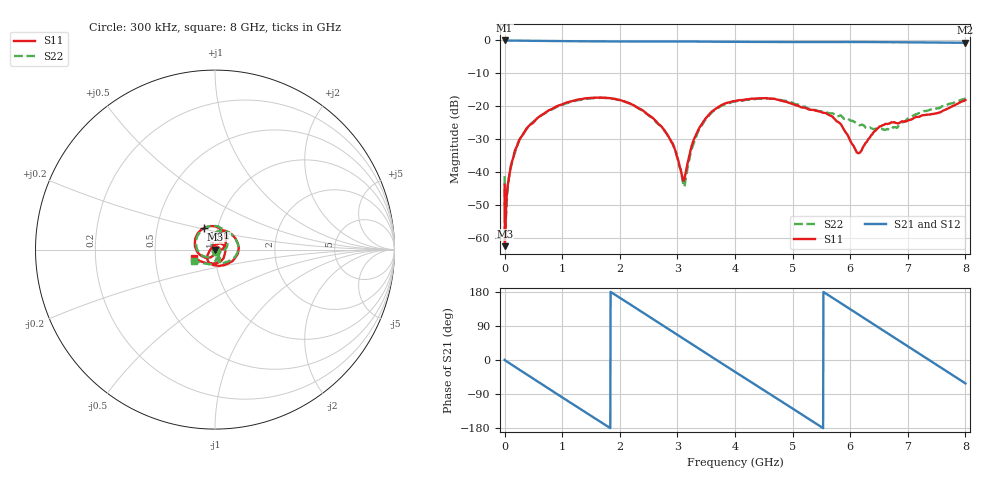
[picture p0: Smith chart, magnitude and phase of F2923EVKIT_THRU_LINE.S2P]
! Integrated Device Technology
! Corporate Headquarters
! 6024 Silver Creek Valley Road
! San Jose, CA 95138  USA
! Phone:  1-408-284-8200
! Toll Free:  1-800-223-1366
! Webpage:  http://www.idt.com/
! Timing and RF Division
! 515 Groton Road, Suite 102
! Westford, MA 01886-6024
! Description: F2923 EVKIT Thru Line
! Frequency:  0.3 MHz to 8 GHz
! Ports:  2 RF, 0 DC
!  EVKit RF Connector J4  = Port 1
!  EVKit RF Connector J5  = Port 2
! Data:  The results below were measured on the F2923 EVKit Thru Line from J4 to J5
!  using a calibrated network analyzer. The reference plane is at
!  the SMA coaxial interfaces.
! Misc:
! Date Measured:  2017-08-14
! Date:  2017-08-14  SPJ
! Note:
!  Integrated Device Technology supplies this data as a sample
!	of measured data. Data was taken at 25 degrees C.
!  Integrated Device Technology reserves the right to change
! 	this data at anytime.
# Hz S dB R 50
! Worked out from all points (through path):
!   1601 points, 300 kHz to 8 GHz, reference 50 ohm
!   highest |S21| = 0.01 dB at 300 kHz (marker M1); lowest = -0.7 dB at 8 GHz (marker M2)
!   group delay of S21, straight-line fit = 271 ps
!   lowest |S11| = -62.6 dB at 5.3 MHz (marker M3), VSWR 1.00, Z = 50.1 - j0.02 ohm
!   |S11| at or under -10 dB: start of sweep to end of sweep
!   |S22| runs from -59.3 to -17.4 dB; largest |S21 - S12| = 0.0061
!   S11 on the Smith chart (normalised r, x): 300 kHz: 1.01, -0.01; 1.61 GHz: 0.86, +0.21; 8 GHz: 0.79, -0.07
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300000  -43.92 -40.7  0.01 0.2  -0.00 0.2  -41.32 -48.5
5299813  -62.63 -15.7  0.00 -0.6  0.00 -0.6  -59.33 55.5
4.529831e7  -45.58 -62.4  -0.01 -4.6  -0.02 -4.6  -46.56 -73.0
9.029662e7  -40.40 -77.5  -0.02 -9.1  -0.03 -9.1  -40.13 -80.4
1.652938e8  -34.50 -88.0  -0.04 -16.6  -0.04 -16.6  -34.82 -95.3
3.952852e8  -26.50 -116.7  -0.08 -39.3  -0.08 -39.3  -26.56 -121.1
8.652676e8  -20.45 -167.9  -0.16 -85.4  -0.16 -85.4  -20.63 -173.9
1.33525e9  -17.88 144.9  -0.24 -131.2  -0.25 -131.2  -17.99 136.4
1.61024e9  -17.39 118.0  -0.27 -157.9  -0.28 -157.9  -17.52 108.9
2.100221e9  -18.71 71.9  -0.29 154.6  -0.29 154.5  -18.73 62.4
2.6702e9  -25.40 16.3  -0.28 99.0  -0.28 99.0  -25.51 -3.5
2.93519e9  -32.22 -3.5  -0.29 73.0  -0.29 73.1  -32.09 -42.9
3.115183e9  -42.53 63.6  -0.30 55.4  -0.30 55.4  -44.56 -138.5
3.440171e9  -24.97 102.1  -0.34 23.5  -0.33 23.5  -25.33 110.4
4.00015e9  -18.43 59.9  -0.41 -31.2  -0.41 -31.1  -18.59 61.7
4.655125e9  -17.74 -7.9  -0.47 -94.6  -0.47 -94.6  -17.75 -0.9
5.3351e9  -21.11 -89.3  -0.48 -160.8  -0.47 -160.8  -20.86 -55.2
5.725085e9  -23.85 -131.9  -0.48 160.8  -0.48 161.0  -22.51 -70.2
6.14007e9  -34.33 137.1  -0.46 120.4  -0.46 120.4  -25.60 -60.9
6.67005e9  -25.34 24.4  -0.52 68.7  -0.52 68.7  -27.12 -56.7
7.335025e9  -22.58 -72.3  -0.60 3.5  -0.61 3.4  -21.42 -108.4
8e9  -18.16 -158.8  -0.70 -61.7  -0.68 -61.8  -17.71 -151.9
